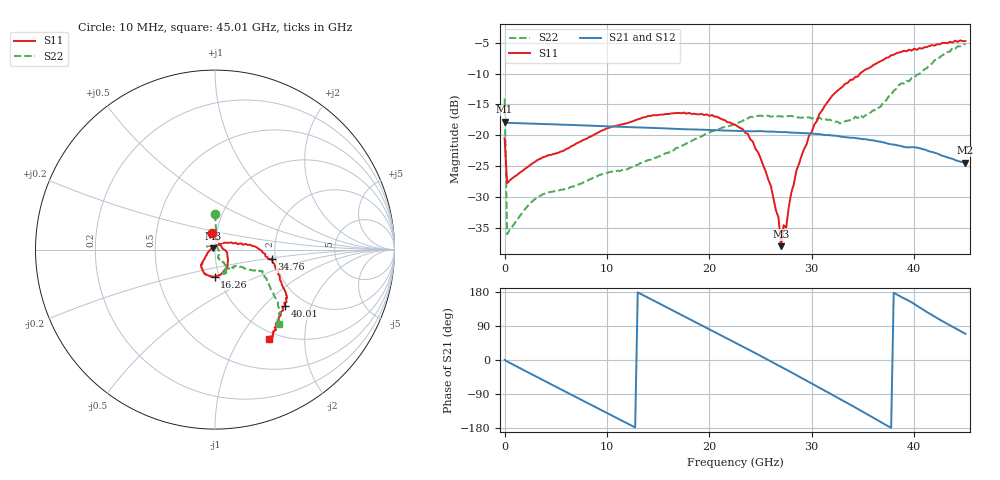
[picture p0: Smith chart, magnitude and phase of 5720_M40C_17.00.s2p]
! Device:  ADRF5720
! Description: 0.5dB LSB GaAs MMIC 6-bit Digital Attenuator
! Frequency:  0.000009 -  40 GHz
! Ports:
!	RF1	= Port 1
!	RF2	= Port 2
! Vdd:  3.3 Volt
! Vss:  -3.3 Volt
! Control:  0/3.3 Volt
! State:  17.00 dB attenuation
! Data:  The device was measured using G-S-G Probes on a matrix board.
!  Data was collected using an calibrated 4 port network analyzer.
!  The reference plane for this measurement is at the launchers.
! Note:  Analog Devices supplies this data as a sample of measured data
!  for this product.  Your particular data for this product may vary.
!  Data was taken at -40 degrees C.
!  Analog Devices reserves the right to change this data at anytime.
# GHZ S DB R 45.0
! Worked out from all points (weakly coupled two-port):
!   181 points, 10 MHz to 45.01 GHz, reference 45 ohm
!   highest |S21| = -17.81 dB at 10 MHz (marker M1); lowest = -24.4 dB at 45.01 GHz (marker M2)
!   lowest |S11| = -38.0 dB at 27.01 GHz (marker M3), VSWR 1.03, Z = 44.1 + j0.659 ohm
!   |S11| at or under -10 dB: start of sweep to 34.72 GHz
!   |S22| runs from -36.0 to -5.2 dB; largest |S21 - S12| = 0.00046
!   S11 on the Smith chart (normalised r, x): 10 MHz: 0.96, +0.18; 16.26 GHz: 0.95, -0.29; 34.76 GHz: 1.90, -0.23; 40.01 GHz: 1.59, -1.34; 45.01 GHz: 0.90, -1.35
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0.01  -20.46 98.5  -17.81 0.2  -17.83 0.2  -14.03 90.1
0.26  -27.77 12.9  -17.99 -3.8  -18.00 -3.9  -36.03 30.8
3.26  -23.97 -8.7  -18.15 -46.1  -18.17 -46.1  -29.94 -32.5
7.76  -20.70 -38.5  -18.40 -108.7  -18.42 -108.7  -27.59 -65.1
15.26  -16.64 -84.5  -18.85 147.0  -18.87 146.9  -23.33 -60.9
16.26  -16.46 -90.6  -18.94 133.1  -18.96 133.0  -22.44 -59.2
20.26  -16.71 -114.0  -19.15 77.4  -19.17 77.3  -19.38 -56.6
22.76  -18.55 -131.3  -19.28 42.5  -19.31 42.4  -18.03 -62.2
24.26  -21.04 -136.6  -19.35 21.6  -19.37 21.5  -17.02 -64.1
25.51  -25.88 -152.3  -19.38 3.4  -19.40 3.2  -16.87 -65.6
26.76  -33.33 160.7  -19.47 -14.6  -19.49 -14.7  -16.88 -67.4
27.01  -37.97 143.8  -19.48 -18.0  -19.50 -18.2  -16.94 -69.3
27.26  -34.58 119.5  -19.48 -21.7  -19.50 -21.9  -17.00 -68.2
27.51  -34.97 74.5  -19.48 -25.4  -19.50 -25.6  -16.87 -69.5
28.01  -29.27 50.2  -19.56 -32.6  -19.58 -32.7  -16.85 -70.5
28.51  -25.68 42.4  -19.59 -39.9  -19.61 -40.1  -17.04 -70.7
30.26  -18.22 17.9  -19.75 -65.8  -19.78 -66.0  -17.11 -69.5
32.01  -13.58 5.6  -20.04 -91.8  -20.06 -92.0  -17.66 -62.0
34.76  -9.91 -9.7  -20.57 -132.9  -20.59 -133.1  -16.76 -44.6
37.76  -7.03 -29.9  -21.46 -178.9  -21.48 -179.1  -13.47 -31.1
40.01  -5.97 -39.0  -21.93 148.0  -21.96 147.8  -10.61 -26.3
45.01  -4.74 -58.9  -24.45 69.1  -24.49 68.9  -5.23 -49.4
